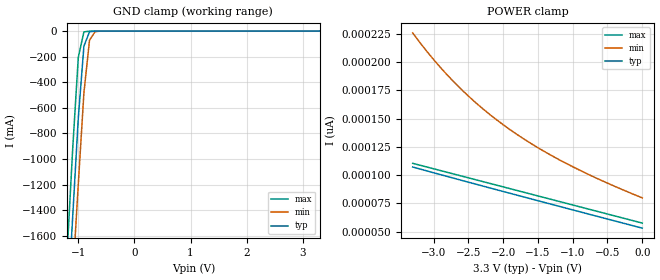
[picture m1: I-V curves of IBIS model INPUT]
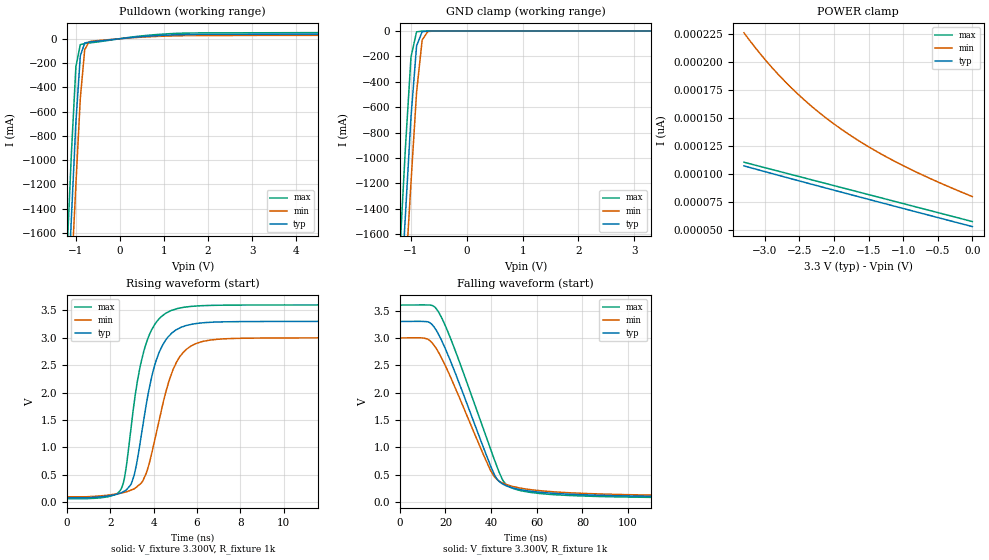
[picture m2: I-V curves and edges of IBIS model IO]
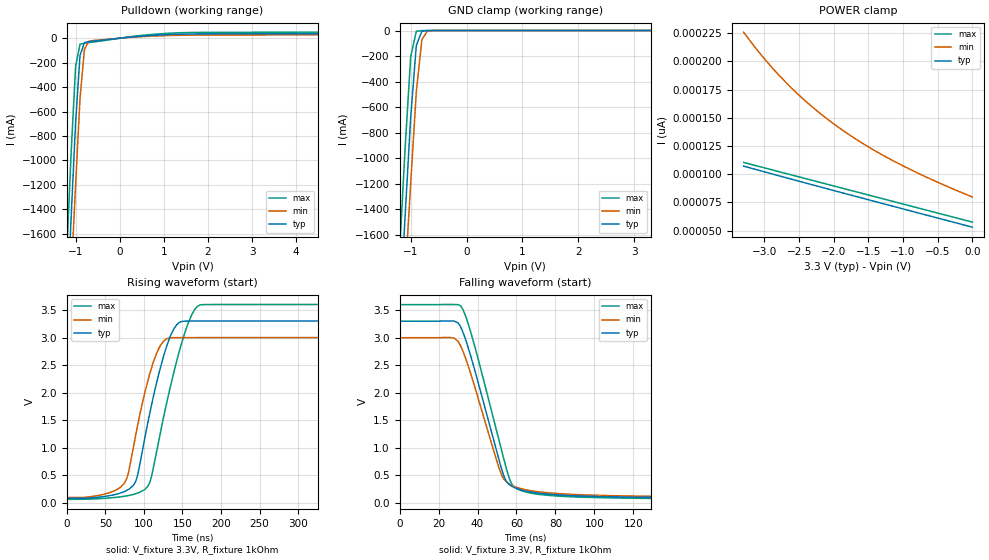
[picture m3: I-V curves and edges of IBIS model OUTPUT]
|   PERICOM SEMICONDUCTOR CORP
|   IBIS Model of PT7C433833
|   Product Family: 7C
|   8 Pin (W) SOIC Package
[IBIS Ver] 4.0
[Comment char] |_char
[File Name] pt7c433833_w_33v.ibs
[File Rev] 1.0
[Source] File originated at Pericom Semiconductor Corp.
[Date] 3/6/2018
[Disclaimer] (C) Copyright PERICOM Semiconductor Corporation
   All rights reserved
  Pericom Semiconductor Corporation hereby grants the user of
  this IBIS model a non-exclusive, nontransferable license to
  use this IBIS model under the following terms.
  This IBIS model is provided on an "AS IS" basis and Pericom
  makes absolutely no warranty with respect to the information
  contained herein. PERICOM DISCLAIMS AND CUSTOMER WAIVES ALL
  WARRANTIES, EXPRESSED OR IMPLIED, INCLUDING WARRANTIES OF
  MERCHANTABILITY OR FITNESS FOR A PARTICULAR PURPOSE. The
  entire risk as to quality and performance is with the customer.
  Accordingly, in no event shall the company be liable for any
  damages, whether in contract or tort, including any lost
  profits or other incidental, consequential, exemplary, or
  punitive damages arising out of the use or application of the
  IBIS model provided in this package. Further, Pericom reserves
  the right to make changes without notice to any product herein
  to improve reliability, function, or design. Pericom does not
  convey any license under patent rights or any other intellectual
  property rights, including those of third parties.
  The user is granted this license only to use the IBIS model
  and is not granted rights to sell, load, rent, lease or license
  the IBIS model in whole or in part, or in modified form to anyone
  other than user. User may modify the IBIS model to suit its specific
  application but rights to derivative works and such modifications
  shall belong to Pericom.
  Pericom is not obligated to provide maintenance or support
  for the licensed IBIS model.
  Contact Pericom at ATTN: APPLICATION ENGINEERING / IBIS MODELS
  Milpitas, CA 95134
[Component] PT7C433833
[Manufacturer] Pericom Semiconductor Corp.
[Package]
|   typ   min   max
R_pkg   0.03093ohm   0.02906ohm   0.03279ohm
L_pkg   2.23473nH   2.04677nH   2.42269nH
C_pkg   0.22955pF   0.20548pF   0.25361pF
[Pin]   signal_name   model_name   R_pin   L_pin   C_pin
1   X1   NC   0.03279   2.42269nH   0.25361pF
2   X2   NC   0.02906   2.04677nH   0.20548pF
3   VBAT   POWER   0.02906   2.04677nH   0.20548pF
4   GND   GND   0.03279   2.26239nH   0.25361pF
5   SDA   IO   0.03279   2.42269nH   0.25361pF
6   SCL   INPUT   0.03279   2.42269nH   0.25361pF
7   SQW/OUT   OUTPUT   0.02906   2.04677nH   0.20548pF
8   VCC   POWER   0.03279   2.42269nH   0.25361pF
| Models and submodels in the file (3): INPUT (Input), IO (I/O_open_drain), OUTPUT (Open_drain)
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|   Model INPUT1
[Model] INPUT
Model_type Input
Vinl = 990mV
Vinh = 2.31V
| variable   typ   min   max
C_comp   1.20pF   1.10pF   1.30pF
[Voltage Range]   3.30V   3.00V   3.60V
[GND Clamp Reference]   0.00V   0.00V   0.00V
[POWER Clamp Reference]  3.30V   3.00V   3.60V
[temperature range]   25   85   -40
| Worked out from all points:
|   GND clamp passes 1 mA (typ) near -0.71 V on its own axis
[GND Clamp]
| Voltage   I(typ)   I(min)  I(max)
-3.3V     -18.52A    -18.19A    -18.98A
-1.2V     -2.228A    -2.673A    -1.742A
-1.1V     -1.452A    -1.934A    -921.1mA
-1V       -678.8mA   -1.196A    -205.4mA
-900mV    -117.9mA   -482.7mA   -6.189mA
-800mV    -5.043mA   -71.03mA   -793.1uA
-700mV    -429.4uA   -4.115mA   -100.8uA
3.3V      53.12pA    87.55pA    52.8pA
[POWER Clamp]
| Voltage   I(typ)   I(min)  I(max)
-3.3V     107.2pA    225.7pA    110.4pA
-3V       102.1pA    202.1pA    105.6pA
-2.7V     97.09pA    181.8pA    100.8pA
-2.4V     92.11pA    164.3pA    96.01pA
-2.2V     88.81pA    154pA      92.8pA
-2V       85.53pA    144.5pA    89.61pA
-1.6V     79.01pA    127.9pA    83.21pA
-1.1V     70.87pA    110.5pA    75.2pA
-600mV    62.79pA    95.66pA    67.2pA
0V        53.11pA    79.85pA    57.6pA
|   Model IO
[Model]  IO
Model_type I/O_open_drain
Vinl = 990mV
Vinh = 2.31V
Vref=3.300V
Vmeas=2.5V
Rref=1k
| variable   typ   min   max
C_comp   1.282pF   1.281pF   1.283pF
[Voltage Range]   3.3000V   3.0000V   3.6000V
[POWER Clamp Reference]  3.3000V   3.0000V   3.6000V
[GND Clamp Reference]   0.0000V   0.0000V   0.0000V
[Pulldown Reference]   0.0000V   0.0000V   0.0000V
[Temperature Range]   25   85   -40
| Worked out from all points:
|   slope of the pulldown table from 0 to 0.495 V, typ, clamps not added: 29 ohm
|   GND clamp passes 1 mA (typ) near -0.71 V on its own axis
|   rising waveform, V_fixture 3.300V, R_fixture 1k: 20-80 % time 955ps typ, 1.12ns min, 872ps max; typ from 0.08 V to 3.3 V
|   falling waveform, V_fixture 3.300V, R_fixture 1k: 20-80 % time 17.7ns typ, 17.9ns min, 18.3ns max; typ from 3.3 V to 0.08 V
[GND Clamp]
| Voltage   I(typ)   I(min)  I(max)
-3.3V     -18.52A    -18.19A    -18.98A
-1.2V     -2.228A    -2.673A    -1.742A
-1.1V     -1.452A    -1.934A    -921.1mA
-1V       -678.8mA   -1.196A    -205.4mA
-900mV    -117.9mA   -482.7mA   -6.189mA
-800mV    -5.043mA   -71.03mA   -793.1uA
-700mV    -429.4uA   -4.115mA   -100.8uA
3.3V      53.12pA    87.55pA    52.8pA
[POWER Clamp]
| Voltage   I(typ)   I(min)  I(max)
-3.3V     107.2pA    225.7pA    110.4pA
-3V       102.1pA    202.1pA    105.6pA
-2.7V     97.09pA    181.8pA    100.8pA
-2.4V     92.11pA    164.3pA    96.01pA
-2.2V     88.81pA    154pA      92.8pA
-2V       85.53pA    144.5pA    89.61pA
-1.6V     79.01pA    127.9pA    83.21pA
-1.1V     70.87pA    110.5pA    75.2pA
-600mV    62.79pA    95.66pA    67.2pA
0V        53.11pA    79.85pA    57.6pA
[Pulldown]
| Voltage   I(typ)   I(min)  I(max)
-3.3V     -18.54A    -18.2A     -18.99A
-1.2V     -2.237A    -2.681A    -1.752A
-1.1V     -1.461A    -1.942A    -931mA
-1V       -689mA     -1.203A    -230.8mA
-900mV    -141.9mA   -492.9mA   -48.95mA
-800mV    -35.18mA   -90.52mA   -40.5mA
-700mV    -27.71mA   -24.93mA   -35.63mA
700mV     22.27mA    16.46mA    30.27mA
1.5V      34.17mA    25.02mA    46.19mA
5.1V      38.86mA    28.69mA    51.8mA
6.6V      48.83mA    36.09mA    65.6mA
[Rising Waveform]
V_fixture = 3.300V
V_fixture_min = 3.00V
V_fixture_max = 3.600V
R_fixture = 1k
|   Time   V(typ)   V(min)   V(max)
0s        79.94mV    97.93mV    63.89mV
2.45ns    163.5mV    160.5mV    209.9mV
2.65ns    202.6mV    178.6mV    440.8mV
2.95ns    324.2mV    220mV      1.347V
3.3ns     899.7mV    306.4mV    2.325V
3.75ns    1.99V      646.8mV    3.006V
4.25ns    2.734V     1.501V     3.345V
5.05ns    3.147V     2.552V     3.53V
7.4ns     3.293V     2.984V     3.596V
30ns      3.3V       3V         3.6V
[Falling Waveform]
V_fixture = 3.300V
V_fixture_min = 3.00V
V_fixture_max = 3.600V
R_fixture = 1k
|   Time   V(typ)   V(min)   V(max)
0s        3.3V       3V         3.6V
12ns      3.296V     2.982V     3.602V
16.5ns    3.101V     2.768V     3.503V
23.5ns    2.441V     2.163V     2.854V
36.5ns    1.011V     878.5mV    1.349V
41.5ns    497.7mV    461.8mV    765.9mV
46.5ns    301.9mV    324.8mV    324.3mV
56ns      207.4mV    236.2mV    186.6mV
140ns     96.49mV    116.5mV    78.24mV
500ns     80.1mV     98.05mV    64.11mV
[Ramp]
| variable   typ   min   max
dV/dt_r   1.9315V/956.66p   1.7400V/1.1253n   2.1200V/876.39p
dV/dt_f   1.9315V/17.725n   1.7400V/17.874n   2.1200V/18.312n
R_load = 1000
|   Model OUTPUT
[Model]  OUTPUT
Model_type Open_drain
Vref = 3.30V
Rref = 1k
Cref =  0
Vmeas = 1.65V
| variable   typ   min   max
C_comp   1.282pF   1.281pF   1.283pF
[Voltage Range]   3.3000V   3.0000V   3.6000V
[POWER Clamp Reference]  3.3000V   3.0000V   3.6000V
[GND Clamp Reference]   0.0000V   0.0000V   0.0000V
[Pullup Reference]   3.3000V   3.0000V   3.6000V
[Pulldown Reference]   0.0000V   0.0000V   0.0000V
[Temperature Range]   25   85   -40
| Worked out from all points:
|   slope of the pulldown table from 0 to 0.495 V, typ, clamps not added: 29 ohm
|   GND clamp passes 1 mA (typ) near -0.71 V on its own axis
|   rising waveform, V_fixture 3.3V, R_fixture 1kOhm: 20-80 % time 30.3ns typ, 27.4ns min, 34.6ns max; typ from 0.08 V to 3.3 V
|   falling waveform, V_fixture 3.3V, R_fixture 1kOhm: 20-80 % time 14.8ns typ, 14.8ns min, 15.5ns max; typ from 3.3 V to 0.08 V
[GND Clamp]
| Voltage   I(typ)   I(min)  I(max)
-3.3V     -18.52A    -18.19A    -18.98A
-1.2V     -2.228A    -2.673A    -1.742A
-1.1V     -1.452A    -1.934A    -921.1mA
-1V       -678.8mA   -1.196A    -205.4mA
-900mV    -117.9mA   -482.7mA   -6.189mA
-800mV    -5.043mA   -71.03mA   -793.1uA
-700mV    -429.4uA   -4.115mA   -100.8uA
3.3V      53.12pA    87.55pA    52.8pA
[POWER Clamp]
| Voltage   I(typ)   I(min)  I(max)
-3.3V     107.1pA    225.7pA    110.4pA
-3V       102.1pA    202.1pA    105.6pA
-2.7V     97.1pA     181.8pA    100.8pA
-2.4V     92.11pA    164.3pA    96.02pA
-2.2V     88.82pA    154pA      92.8pA
-2V       85.53pA    144.5pA    89.61pA
-1.6V     79.01pA    127.9pA    83.2pA
-1.1V     70.88pA    110.5pA    75.2pA
-600mV    62.79pA    95.66pA    67.2pA
0V        53.12pA    79.85pA    57.6pA
[Pulldown]
|Voltage   I(typ)   I(min)   I(max)
-3.3V     -18.54A    -18.2A     -18.99A
-1.2V     -2.237A    -2.681A    -1.752A
-1.1V     -1.461A    -1.942A    -931mA
-1V       -689mA     -1.203A    -230.8mA
-900mV    -141.9mA   -492.9mA   -48.95mA
-800mV    -35.18mA   -90.52mA   -40.5mA
-700mV    -27.71mA   -24.93mA   -35.63mA
700mV     22.27mA    16.46mA    30.27mA
1.5V      34.17mA    25.02mA    46.19mA
5.1V      38.86mA    28.69mA    51.8mA
6.6V      48.83mA    36.09mA    65.6mA
[Rising Waveform]
V_fixture = 3.3V
V_fixture_min = 3.0V
V_fixture_max = 3.6V
R_fixture = 1kOhm
C_fixture = 0F
|   Time   V(typ)   V(min)   V(max)
0s        79.94mV    97.93mV    63.89mV
75ns      206mV      365.8mV    120.3mV
80ns      243.4mV    551.9mV    132.6mV
91ns      457.2mV    1.35V      173.8mV
105ns     1.45V      2.211V     300.7mV
121ns     2.434V     2.847V     1.253V
138ns     3.136V     2.998V     2.329V
157ns     3.299V     3V         3.248V
170ns     3.3V       3V         3.573V
420ns     3.3V       3V         3.6V
[Falling Waveform]
V_fixture = 3.3V
V_fixture_min = 3.0V
V_fixture_max = 3.6V
R_fixture = 1kOhm
C_fixture = 0F
|   Time   V(typ)   V(min)   V(max)
0s        3.3V       3V         3.6V
28ns      3.301V     2.993V     3.602V
31.5ns    3.183V     2.838V     3.57V
37.5ns    2.547V     2.235V     2.982V
50.5ns    845.6mV    692.1mV    1.21V
54ns      446.7mV    409.1mV    729.5mV
58.5ns    283.9mV    302mV      302.9mV
68ns      192mV      217.6mV    171.9mV
150ns     92.47mV    111.4mV    75.04mV
520ns     79.98mV    97.95mV    63.97mV
[Ramp]
| variable   typ   min   max
dV/dt_r  1.9309V/30.267n   1.7380V/27.305n   2.1200V/34.567n
dV/dt_f  1.9309V/14.844n   1.7380V/14.774n   2.1200V/15.499n
R_load = 1000
